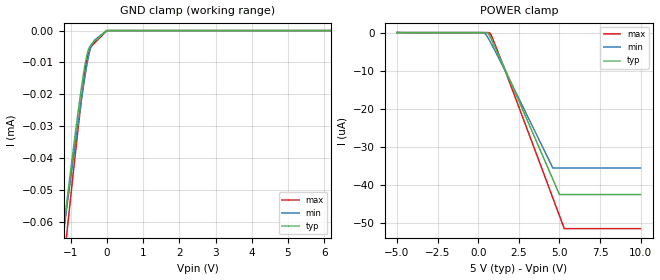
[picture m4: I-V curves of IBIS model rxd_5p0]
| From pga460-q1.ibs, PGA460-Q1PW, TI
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|   rxd_5p0 Model
[Model]   rxd_5p0
Model_type   Input
Vinl = 1.5
Vinh = 3.5
|   typ   min   max
|   (nom PVT)   (fast PVT)   (slow PVT)
C_comp   1.786e-13   1.763e-13   1.934e-13
| Where nom  PVT is Nominal Process, 5V, 27C
|   Fast PVT is Strong Process,  5.3V, -40C
|   Slow PVT is Weak Process,   4.6V, 125C
[Voltage Range]   5   4.6   5.3
|Junction Temperature
[Temperature Range]   27   125   -40
[Power Clamp Reference]   5   4.6   5.3
[GND Clamp Reference]   0   0   0
[GND Clamp]
|   Voltage   I(typ)   I(min)   I(max)
-5V       -442.2uA   -407.7uA   -501uA
-1.245V   -66.49uA   -67.5uA    -78.63uA
-1.154V   -57.97uA   -59.57uA   -68.71uA
-1.09V    -51.96uA   -53.97uA   -61.71uA
-929.6mV  -37.26uA   -40.2uA    -44.51uA
-717.6mV  -18.96uA   -22.72uA   -22.85uA
-616.9mV  -11.44uA   -15.07uA   -13.74uA
-542.7mV  -7.236uA   -10.07uA   -8.504uA
-464.4mV  -4.87uA    -5.959uA   -5.592uA
-386.2mV  -3.836uA   -3.714uA   -4.414uA
-4.4mV    -43.48nA   0A         -26.35nA
10V       0A         0A         0A
[POWER Clamp]
|   Voltage   I(typ)   I(min)   I(max)
-5V       2.216nA    361.7pA    59.52nA
290mV     12.43pA    -12.67nA   15.96pA
414.2mV   -289.5pA   -230.6nA   14.81pA
549.1mV   -46.61nA   -981.6nA   -44.63pA
704mV     -842nA     -2.115uA   -88.86nA
795mV     -1.584uA   -2.829uA   -668.9nA
915mV     -2.645uA   -3.798uA   -1.819uA
1.413V    -7.333uA   -7.963uA   -7.232uA
4.6V      -38.59uA   -35.6uA    -43.5uA
5.005V    -42.59uA   -35.6uA    -48.14uA
5.303V    -42.59uA   -35.6uA    -51.55uA
10V       -42.59uA   -35.6uA    -51.55uA
